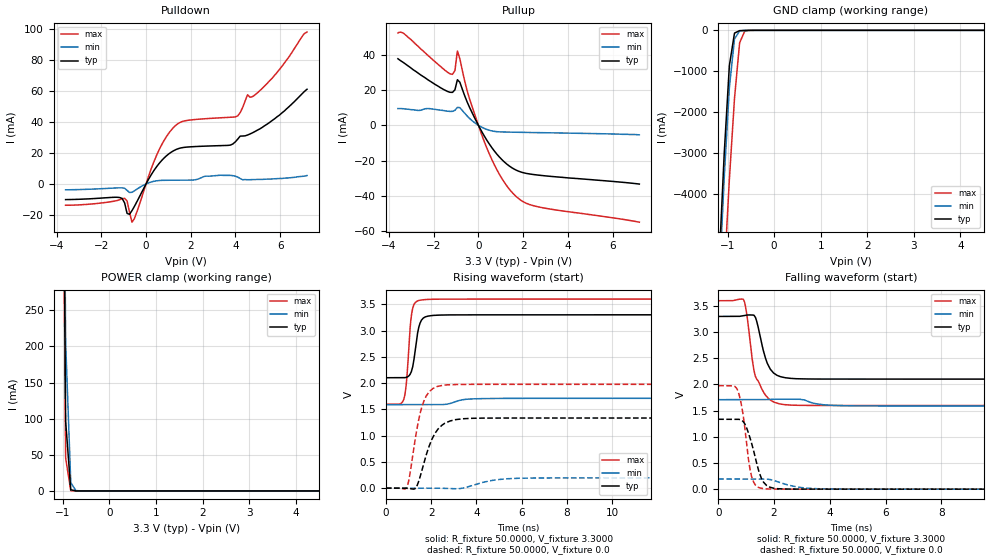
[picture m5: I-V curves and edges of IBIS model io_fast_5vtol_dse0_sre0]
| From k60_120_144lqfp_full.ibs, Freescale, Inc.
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[Model]  io_fast_5vtol_dse0_sre0
|   Model io_fast_5vtol_dse0_sre0
| Library cells for typ/min/max conditions are connected as defined below:
|  pad - External Pad
|  ipp_do - Core Input
|  ipp_obe - Output Buffer Enable
|  esd_boost - vdd_s_3v
|  esd_bus - vdd_s_3v
|  ipp_ame - vss_s_lv
|  ipp_dse - vss_s_lv
|  ipp_ina40a_5vtol - NC
|  ipp_ina40b_5vtol - NC
|  ipp_ina_5vtol - NC
|  ipp_ina_mux_3v - NC
|  ipp_ind - NC
|  ipp_ind_3v - NC
|  ipp_pue - vss_s_lv
|  ipp_sre - vss_s_lv
|  tie_3v - vdd_s_3v
|  tie_hi - vdd_s_lv
|  vbuf_3v - vdd_s_3v
|  vdd_bulk_lv - vdd_s_lv
|  vdd_s_3v - vdd_s_3v
|  vdd_s_lv - vdd_s_lv
|  vss_bulk - vss_s_3v
|  vss_s_3v - vss_s_3v
|  vss_s_lv - vss_s_lv
| All other pins connected to ground
Model_type I/O
Polarity   Non-Inverting
Enable   Active-High
Vinl =   1.1550V
Vinh =   2.3100V
Vmeas =  1.6500V
Cref =   25.0000pF
Rref =   50.0000
Vref =   0.0V
C_comp   4.6080pF   4.5393pF   4.8314pF
[Temperature Range]   25.0000   0.1250k   -40.0000
[Voltage Range]   3.3000V   1.7100V   3.6000V
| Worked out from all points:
|   slope of the pulldown table from 0 to 0.495 V, typ, clamps not added: 43 ohm
|   slope of the pullup table from 0 to 0.495 V, typ, clamps not added: 46.1 ohm
|   GND clamp passes 1 mA (typ) near -0.54 V on its own axis
|   POWER clamp passes 1 mA (typ) near -0.79 V on its own axis
|   rising waveform, R_fixture 50.0000, V_fixture 3.3000: 20-80 % time 255ps typ, 573ps min, 200ps max; typ from 2.1 V to 3.3 V
|   rising waveform, R_fixture 50.0000, V_fixture 0.0: 20-80 % time 665ps typ, 1.09ns min, 506ps max; typ from 0 V to 1.33 V
|   falling waveform, R_fixture 50.0000, V_fixture 3.3000: 20-80 % time 373ps typ, 585ps min, 433ps max; typ from 3.3 V to 2.1 V
|   falling waveform, R_fixture 50.0000, V_fixture 0.0: 20-80 % time 418ps typ, 830ps min, 293ps max; typ from 1.33 V to 0 V
[Pulldown]
|Voltage   I(typ)   I(min)   I(max)
-3.6V     -10.1mA    -3.79mA    -13.73mA
-1.29V    -8.593mA   -2.576mA   -10.67mA
-960mV    -12.21mA   -2.816mA   -9.278mA
-850mV    -18.97mA   -4.144mA   -11mA
-630mV    -17.18mA   -5.369mA   -24.63mA
470mV     11.04mA    1.994mA    18.36mA
1.24V     21.41mA    2.381mA    36.48mA
4.1V      28.81mA    4.4mA      43.8mA
4.54V     31.46mA    2.7mA      57.37mA
4.76V     32.88mA    2.8mA      56.16mA
5.64V     40.8mA     3.2mA      68mA
7.2V      60.9mA     5.4mA      97.7mA
[Pullup]
|Voltage   I(typ)   I(min)   I(max)
-3.6V     37.7mA     9.5mA      52.3mA
-3.36V    35.6mA     9.4mA      52.2mA
-1.27V    18.7mA     7.87mA     29.17mA
-1.05V    20.11mA    8.49mA     31.01mA
-940mV    25.83mA    10.14mA    42.08mA
-830mV    24.4mA     9.99mA     37.76mA
-390mV    9.99mA     3.842mA    14.73mA
380mV     -8.486mA   -2.363mA   -12.95mA
1.04V     -19.31mA   -3.754mA   -29.93mA
1.81V     -26.05mA   -3.958mA   -41.62mA
2.8V      -28.38mA   -4.169mA   -46.51mA
7.2V      -33.28mA   -5.4mA     -54.88mA
[GND_clamp]
|Voltage   I(typ)   I(min)   I(max)
-3.6V     -73.34A    -73.38A    -74.77A
-1.18V    -5.66A     -6.204A    -8.642A
-1.07V    -2.998A    -3.591A    -5.955A
-960mV    -859.3mA   -1.396A    -3.637A
-850mV    -67.61mA   -209.6mA   -1.663A
-740mV    -7.668mA   -15.82mA   -304.8mA
-630mV    -2.587mA   -2.146mA   -18.83mA
-520mV    -662.1uA   -523uA     -1.741mA
7.2V      0A         0A         0A
[POWER_clamp]
|Voltage   I(typ)   I(min)   I(max)
-3.6V     45.85A     45.45A     46.17A
-1.05V    1.004A     1.14A      941.6mA
-940mV    96.57mA    206.1mA    45.73mA
-830mV    1.646mA    11.48mA    218.1uA
-720mV    22.84uA    474.3uA    919.1nA
-610mV    316.6nA    19.24uA    4.178nA
7.2V      0A         0A         0A
[Ramp]
| variable   typ   min   max
dV/dt_r  0.8010/0.6647n   0.1167/1.0916n   1.1859/0.5065n
dV/dt_f  0.7186/0.3727n   72.4038m/0.5845n   1.2013/0.4330n
R_load = 50.0000
[Rising Waveform]
R_fixture= 50.0000
V_fixture= 3.3000
V_fixture_min= 1.7100
V_fixture_max= 3.6000
|time   V(typ)   V(min)   V(max)
0s        2.102V     1.589V     1.597V
795.1ps   2.103V     1.589V     1.695V
926.1ps   2.111V     1.589V     2.09V
1.07ns    2.167V     1.589V     3.039V
1.136ns   2.232V     1.589V     3.311V
1.245ns   2.457V     1.589V     3.499V
1.507ns   3.138V     1.59V      3.578V
2.541ns   3.297V     1.591V     3.598V
4.285ns   3.3V       1.704V     3.599V
20ns      3.3V       1.71V      3.6V
[Rising Waveform]
R_fixture= 50.0000
V_fixture= 0.0
V_fixture_min= 0.0
V_fixture_max= 0.0
|time   V(typ)   V(min)   V(max)
0s        1.032nV    107.1nV    632.6pV
921.7ps   -2.761mV   -624.3nV   12.95mV
1.03ns    -8.03mV    1.122uV    183.8mV
1.333ns   10.37mV    12.46uV    1.029V
1.66ns    444.4mV    382.1uV    1.637V
2.024ns   921.1mV    229uV      1.876V
2.477ns   1.197V     -2.91mV    1.956V
3.372ns   1.32V      -1.83mV    1.975V
5.867ns   1.335V     187.5mV    1.976V
20ns      1.335V     194.5mV    1.976V
[Falling Waveform]
R_fixture= 50.0000
V_fixture= 3.3000
V_fixture_min= 1.7100
V_fixture_max= 3.6000
|time   V(typ)   V(min)   V(max)
0s        3.3V       1.71V      3.6V
906.2ps   3.314V     1.71V      3.624V
1.011ns   3.325V     1.71V      3.393V
1.217ns   3.327V     1.71V      2.494V
1.328ns   3.287V     1.709V     2.161V
1.762ns   2.403V     1.713V     1.756V
1.984ns   2.22V      1.718V     1.668V
2.176ns   2.161V     1.719V     1.632V
4.76ns    2.103V     1.592V     1.599V
20ns      2.102V     1.589V     1.598V
[Falling Waveform]
R_fixture= 50.0000
V_fixture= 0.0
V_fixture_min= 0.0
V_fixture_max= 0.0
|time   V(typ)   V(min)   V(max)
0s        1.335V     194.5mV    1.977V
699.3ps   1.335V     194.5mV    1.885V
890.8ps   1.295V     194.6mV    1.429V
1.088ns   1.067V     194.5mV    559mV
1.198ns   877.1mV    194.2mV    241.3mV
1.331ns   598.7mV    194mV      79.77mV
1.596ns   162.9mV    194.6mV    11.1mV
1.97ns    19.67mV    169.4mV    1.889mV
3.757ns   538.4uV    5.537mV    552.6uV
20ns      186uV      36.48uV    200.8uV
